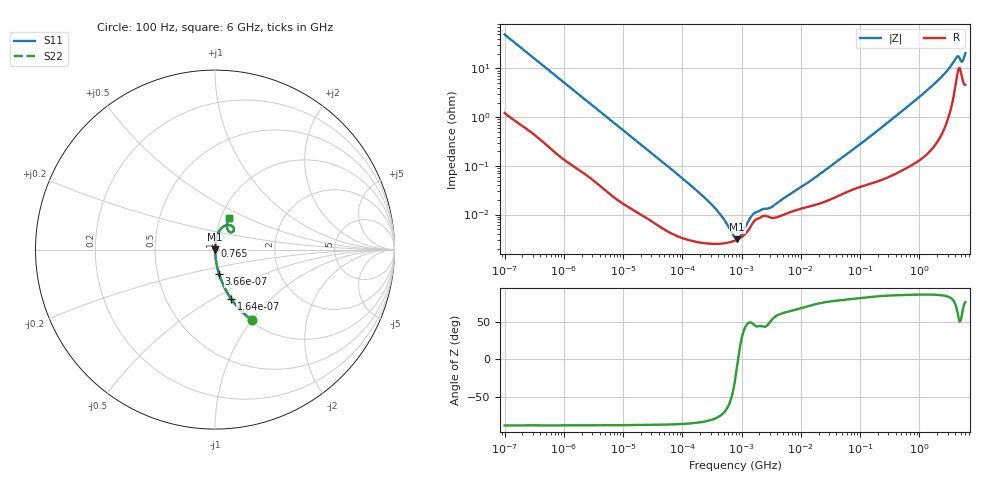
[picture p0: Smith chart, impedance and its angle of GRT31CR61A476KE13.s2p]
!Murata Part Number: GRT31CR61A476KE13
!These Parameters are Measured in Series Mode Connection
!Data Generated on Jun 19, 2026
!  o--ll--o
!Port1  Port2
!  o------o
!Operation Temp=25[degC], DC Bias Voltage=0[V]
!Freq. Start=100[Hz] Stop=6[GHz] 401[Steps]
# Hz S RI R 50
!Freq.(Hz) S11(Real) S11(Imag) S21(Real) S21(Imag) S12(Real) S12(Imag) S22(Real) S22(Imag)
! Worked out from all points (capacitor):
!   401 points, 100 Hz to 6 GHz, reference 50 ohm
!   read as one part in series: C = 31.8 uF near 109 Hz
!   lowest |Z| = 3.08 mohm at 847.2 kHz (marker M1)
!   series resonance near 872.1 kHz, so ESL is about 1 nH
!   S11 on the Smith chart (normalised r, x): 100 Hz: 1.02, -1.00; 164 Hz: 1.02, -0.61; 366 Hz: 1.01, -0.28; 765 MHz: 1.00, +0.04; 6 GHz: 1.09, +0.40
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100  0.2049 -0.3916  0.7951 0.3916  0.7951 0.3916  0.2049 -0.3916
164  0.0918 -0.2764  0.9082 0.2764  0.9082 0.2764  0.0918 -0.2764
366  0.0225 -0.1354  0.9775 0.1354  0.9775 0.1354  0.0225 -0.1354
784  0.00598 -0.0653  0.994 0.0653  0.994 0.0653  0.00598 -0.0653
2008  0.00143 -0.026  0.9986 0.026  0.9986 0.026  0.00143 -0.026
40335  5.97e-05 -0.00137  0.9999 0.00137  0.9999 0.00137  5.97e-05 -0.00137
184852  2.71e-05 -0.000292  1 0.000292  1 0.000292  2.71e-05 -0.000292
432798  2.52e-05 -9.94e-05  1 9.94e-05  1 9.94e-05  2.52e-05 -9.94e-05
495019  2.56e-05 -7.83e-05  1 7.83e-05  1 7.83e-05  2.56e-05 -7.83e-05
774597  2.92e-05 -1.57e-05  1 1.57e-05  1 1.57e-05  2.92e-05 -1.57e-05
847162  3.06e-05 -3.8e-06  1 3.8e-06  1 3.8e-06  3.06e-05 -3.8e-06
1449809  5.87e-05 6.89e-05  0.9999 -6.89e-05  0.9999 -6.89e-05  5.87e-05 6.89e-05
2268635  9.23e-05 9.07e-05  0.9999 -9.07e-05  0.9999 -9.07e-05  9.23e-05 9.07e-05
3103719  8.66e-05 0.000109  0.9999 -0.000109  0.9999 -0.000109  8.66e-05 0.000109
1.555665e7  0.000152 0.0005  0.9998 -0.0005  0.9998 -0.0005  0.000152 0.0005
3.124326e8  0.000665 0.0082  0.9993 -0.0082  0.9993 -0.0082  0.000665 0.0082
7.650043e8  0.00144 0.0198  0.9986 -0.0198  0.9986 -0.0198  0.00144 0.0198
2.240541e9  0.00767 0.0617  0.9923 -0.0617  0.9923 -0.0617  0.00767 0.0617
3.352442e9  0.0246 0.1045  0.9754 -0.1045  0.9754 -0.1045  0.0246 0.1045
4.193612e9  0.0721 0.1378  0.9279 -0.1378  0.9279 -0.1378  0.0721 0.1378
5.245841e9  0.0748 0.1032  0.9252 -0.1032  0.9252 -0.1032  0.0748 0.1032
6e9  0.0782 0.177  0.9218 -0.177  0.9218 -0.177  0.0782 0.177
